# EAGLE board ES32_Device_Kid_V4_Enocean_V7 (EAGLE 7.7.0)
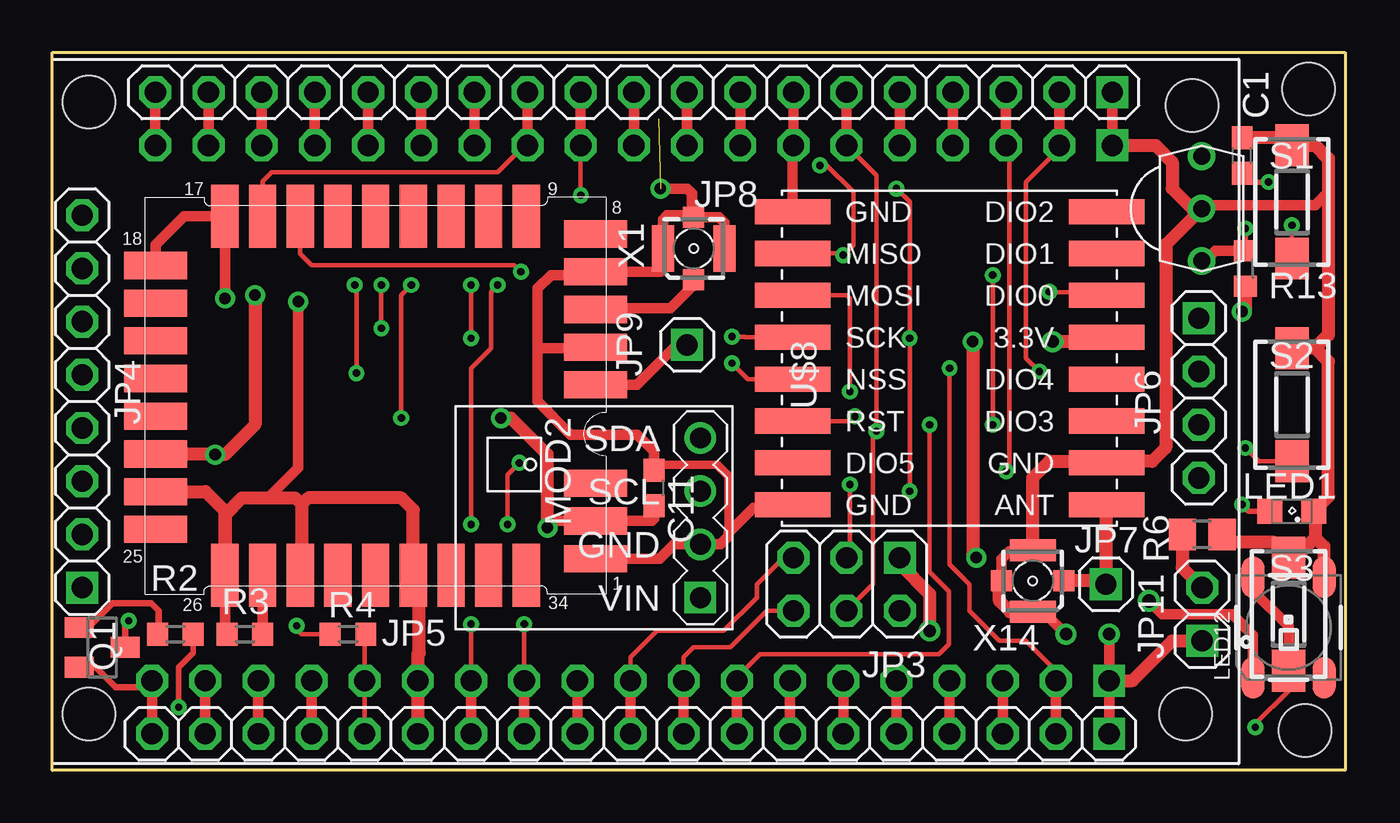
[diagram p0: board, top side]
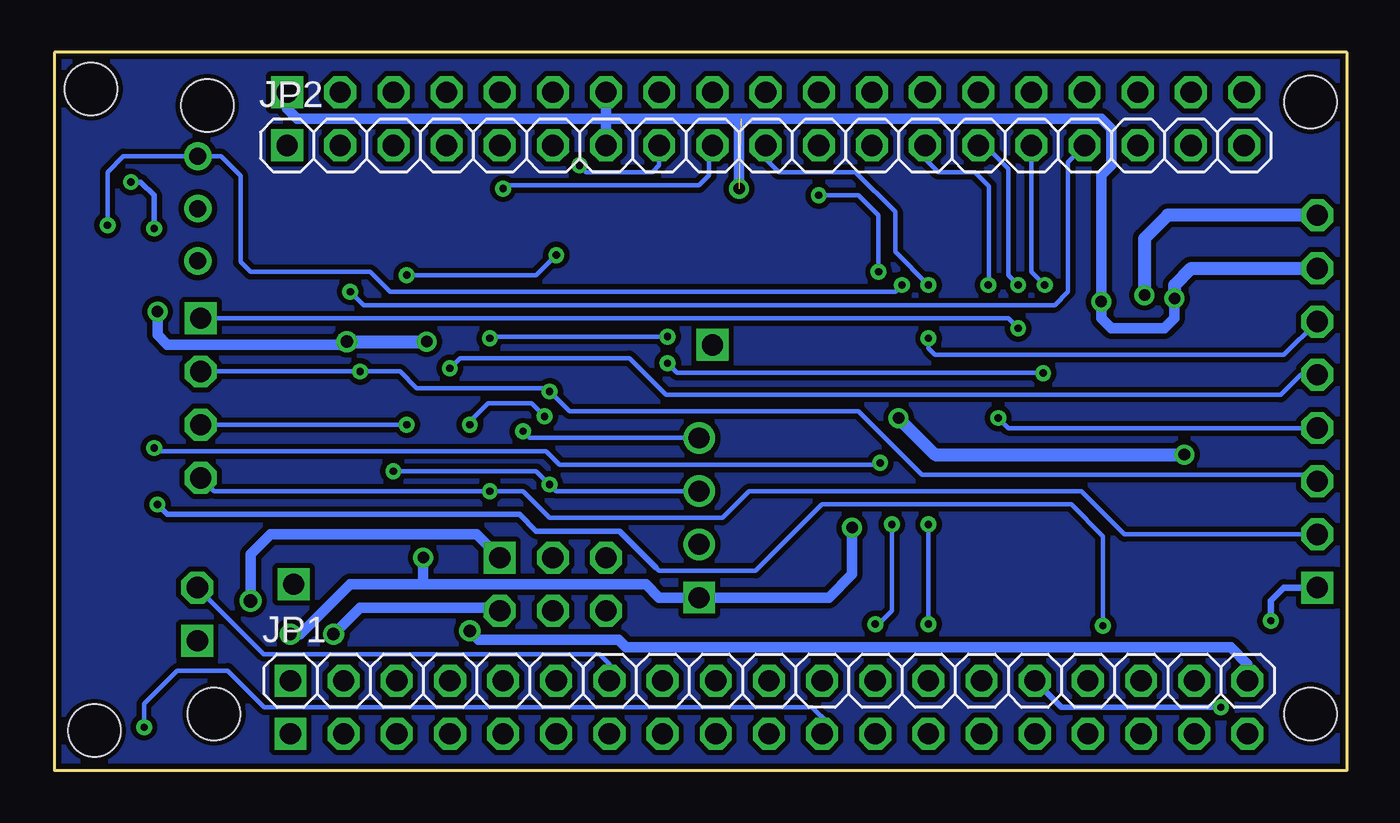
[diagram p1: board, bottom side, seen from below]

Size 61.75 x 34.29 mm. Coordinates in mm from the lower left corner, seen from the top.
Outline: 0,34.29 61.75,34.29 61.75,0 0,0 0,34.29
Copper layers (1*16): Top 0.035mm / dielectric 1.5mm / Bottom 0.035mm
Design rules "default *": minimum track width 6mil, minimum drill 0.35mm, track to track 6mil, track to pad 6mil, pad to pad 6mil, via to via 6mil, smd to smd 6mil, copper to edge 10mil, drill to drill 6mil, minimum pad ring 10mil, minimum via ring 8mil, stop-mask expansion 4mil, vias tented up to drill 0mil, thermal gap 10mil
Net classes: 1 pwr: width 0.25 mm, clearance 0.152 mm to class 0, clearance 0.152 mm
Holes 2.5 mm at 54.13,2.7 59.85,1.91 60.01,32.54 1.75,31.91 54.45,31.75 1.75,2.7

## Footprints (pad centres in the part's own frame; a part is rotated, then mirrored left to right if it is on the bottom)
STM300(C)_TCM300(C)_FOOTPRINT = smd 3 x 1.3: 1 21.5,1.7; 2 21.5,3.5; 3 21.5,5.3; 4 21.5,10; 5 21.5,11.8; 6 21.5,13.6; 7 21.5,15.4; 8 21.5,17.2; 18 0.5,15.7; 19 0.5,13.9; 20 0.5,12.1; 21 0.5,10.3; 22 0.5,8.5; 23 0.5,6.7; 24 0.5,4.9; 25 0.5,3.1 | smd 1.3 x 3: 9 18.2,18.05; 10 16.4,18.05; 11 14.6,18.05; 12 12.8,18.05; 13 11,18.05; 14 9.2,18.05; 15 7.4,18.05; 16 5.6,18.05; 17 3.8,18.05; 26 3.8,0.9; 27 5.6,0.9; 28 7.4,0.9; 29 9.2,0.9; 30 11,0.9; 31 12.8,0.9; 32 14.6,0.9; 33 16.4,0.9; 34 18.2,0.9
C0603 = smd 1.1 x 1: 1 -0.85,0; 2 0.85,0
1X19-S = drill 1.016 square: 1 -22.86,0 | drill 1.016 octagon: 2 -20.32,0; 3 -17.78,0; 4 -15.24,0; 5 -12.7,0; 6 -10.16,0; 7 -7.62,0; 8 -5.08,0; 9 -2.54,0; 10 0,0; 11 2.54,0; 12 5.08,0; 13 7.62,0; 14 10.16,0; 15 12.7,0; 16 15.24,0; 17 17.78,0; 18 20.32,0; 19 22.86,0
2X03 = drill 1.016 square: 1 -2.54,-1.27 | drill 1.016 octagon: 2 -2.54,1.27; 3 0,-1.27; 4 0,1.27; 5 2.54,-1.27; 6 2.54,1.27
1X08-S = drill 1.016 square: 1 -8.89,0 | drill 1.016 octagon: 2 -6.35,0; 3 -3.81,0; 4 -1.27,0; 5 1.27,0; 6 3.81,0; 7 6.35,0; 8 8.89,0
1X04-S = drill 1.016 square: 1 -3.81,0 | drill 1.016 octagon: 2 -1.27,0; 3 1.27,0; 4 3.81,0
1X01-S = drill 1.016 square: 1 0,0
1X02-S = drill 1.016 square: 1 -1.27,0 | drill 1.016 octagon: 2 1.27,0
SML0805 = smd 1.2 x 1.2: A 1.05,0; C -1.05,0
WS2812B = smd 2 x 1.1: 1 -2.4,1.7; 2 -2.4,-1.7; 3 2.4,-1.7; 4 2.4,1.7
TEMP-HUM-PRES-BME280 = drill 1 square: 1 -5.08,3.81 | drill 1: 2 -5.08,1.27; 3 -5.08,-1.27; 4 -5.08,-3.81
SOT23 = smd 1 x 1.4: 1 -0.95,-1.1; 2 0.95,-1.1; 3 0,1.1
R0603 = smd 1 x 1.1: 1 -0.85,0; 2 0.85,0
R0805 = smd 1.3 x 1.5: 1 -0.95,0; 2 0.95,0
DTSM-3 = smd 2 x 1.6: 1 -2.7,0; 2 2.7,0
TSOP18XX = drill 0.813: GND -0.001,-0.027; OUT -2.501,-0.027; VCC 2.499,-0.027
WIRELESS-LORA-RFM95W#SMD = smd 3.6 x 1.2: A1 -7.5,7; A2 -7.5,5; A3 -7.5,3; A4 -7.5,1; A5 -7.5,-1; A6 -7.5,-3; A7 -7.5,-5; A8 -7.5,-7; B1 7.5,7; B2 7.5,5; B3 7.5,3; B4 7.5,1; B5 7.5,-1; B6 7.5,-3; B7 7.5,-5; B8 7.5,-7
734120110 = smd 1 x 1: 1 0,-1.5; S@1 0,1.5 | smd 1.05 x 2.2: S@2 -1.475,0; S@3 1.475,0

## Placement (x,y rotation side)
BRD1  STM300(C)_TCM300(C)_DEVICE  [STM300(C)_TCM300(C)_FOOTPRINT]  4.45,8.41 0 top
C1  100n  [C0603]  56.83,29.37 90 top
C11  100nF  [C0603]  28.73,13.49 270 top
JP1  [1X19-S]  27.62,4.29 0 bottom
JP2  [1X19-S]  27.78,29.84 0 bottom
JP3  [2X03]  37.94,8.89 180 top
JP4  [1X08-S]  1.43,17.62 90 top
JP5  [1X19-S]  27.62,1.75 180 top
JP6  [1X04-S]  54.77,17.78 270 top
JP7  [1X01-S]  50.32,8.89 0 top
JP8  [1X19-S]  27.78,32.38 180 top
JP9  [1X01-S]  30.32,20.32 0 top
JP11  [1X02-S]  54.93,7.46 90 top
LED1  [SML0805]  59.21,12.38 180 top
LED12  WS2812B  [WS2812B]  59.05,6.83 90 top
MOD2  TEMP-HUM-PRES-BME280  [TEMP-HUM-PRES-BME280]  25.88,12.06 180 top
Q1  BSS84/IRLML2244  [SOT23]  2.38,5.87 270 top
R2  2K2  [R0603]  5.87,6.51 180 top
R3  10K / 0603  [R0603]  9.21,6.51 0 top
R4  470R  [R0603]  14.13,6.51 0 top
R6  470R  [R0805]  54.93,11.27 180 top
R13  100R  [R0603]  56.99,23.97 270 top
S1  DTSM-3  [DTSM-3]  59.21,27.15 270 top
S2  DTSM-3  [DTSM-3]  59.21,17.46 270 top
S3  DTSM-3  [DTSM-3]  59.05,7.46 270 top
U$5  TSOP1833  [TSOP18XX]  54.93,26.83 270 top
U$8  WIRELESS-LORA-RFM95W#SMD  [WIRELESS-LORA-RFM95W#SMD]  42.86,19.68 0 top
X1  734120110  [734120110]  30.64,24.92 0 top
X14  734120110  [734120110]  46.83,9.05 90 top

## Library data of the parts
BRD1 = STM300_TCM300_Eagle_Footprint
C1 = rcl; SPICEPREFIX: C
C11 = rcl@1
JP1-JP9 JP11 = pinhead-2
LED1 = led
LED12 = WS2812
MOD2 = diy-modules2
Q1 = transistor-small-signal
R2-R4 R6 R13 = rcl; SPICEPREFIX: R
S1-S3 = switch-tact
U$5 = tsop
U$8 = diy-modules
X1 X14 = con-coax

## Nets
+3V3: BRD1.2 BRD1.23 C11.2 JP1.1 JP4.8 JP5.1 JP11.1 MOD2.1 R13.2 U$8.B4
+5V: JP1.19 JP3.1 JP5.19 LED12.1 Q1.2
ENORES: BRD1.27 R3.2
GND [pwr]: BRD1.1 BRD1.5 BRD1.7 BRD1.17 BRD1.18 BRD1.24 BRD1.26 BRD1.28 BRD1.31 C1.2 C11.1 JP1.14 JP2.1 JP2.7 JP3.2 JP4.7 JP5.14 JP8.1 JP8.7 LED1.C LED12.3 MOD2.2 R3.1 R6.1 S1.1 S2.1 S3.1 U$5.GND U$8.A1 U$8.A8 U$8.B7 X1.S@1 X1.S@2 X1.S@3 X14.S@1 X14.S@2 X14.S@3
GP00_T1: JP2.14 JP6.1 JP8.14
GP01_TX0*: JP2.4 JP8.4
GP02_T2: JP2.15 JP8.15 U$8.A5
GP03_RX0*: JP2.5 JP8.5
GP04_T0: JP2.13 JP4.4 JP8.13
GP05_SS: JP2.10 JP4.6 JP8.10
GP06_SPI*: JP2.19 JP8.19
GP07_SPI*: JP2.18 JP8.18
GP08_SPI*: JP2.17 JP8.17
GP9_SPI*: JP1.16 JP5.16
GP10_SPI*: JP1.17 JP5.17
GP11_SPI*: JP1.18 JP5.18
GP12_T5: JP1.13 JP5.13 S1.2 U$5.OUT
GP13_ADC2-4: JP1.15 JP5.15 R2.1 R4.2
GP14_T6: JP1.12 JP5.12 S2.2
GP15_T3: JP2.16 JP8.16 U$8.B3
GP16_RX2: BRD1.16 JP2.12 JP8.12
GP17_TX2: BRD1.15 JP2.11 JP8.11
GP18_CLK: JP2.9 JP4.2 JP6.4 JP8.9 U$8.A4
GP19_MISO: JP2.8 JP6.3 JP8.8 U$8.A2
GP21_I2C-SDA: JP2.6 JP3.4 JP8.6 MOD2.4
GP22_I2C-CLK: JP2.3 JP3.3 JP8.3 MOD2.3
GP23_MOSI: JP2.2 JP4.3 JP6.2 JP8.2 U$8.A3
GP25_DAC1: JP1.9 JP3.6 JP5.9
GP26_DAC2: JP1.10 JP3.5 JP5.10
GP27_T7: JP1.11 JP5.11 LED12.4 S3.2
GP32_T9: JP1.7 JP5.7 JP11.2 R6.2
GP33_T8: JP1.8 JP5.8 U$8.A6
GP34_IN*: JP1.5 JP5.5
GP35_IN*: JP1.6 JP5.6
GP36_IN*: JP1.3 JP5.3
GP39_IN*: JP1.4 JP5.4
N$1: LED1.A R4.1
N$2: JP4.1 Q1.3
N$3: Q1.1 R2.2
N$8: JP7.1 U$8.B8 X14.1
N$9: C1.1 R13.1 U$5.VCC
RESET: JP1.2 JP4.5 JP5.2
RF50R: BRD1.6 X1.1
RFWIPE: BRD1.4 JP9.1

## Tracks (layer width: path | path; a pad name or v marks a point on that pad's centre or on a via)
+3V3  (via drill 0.55, 0.6)
  Top 0.508: U$8.B4 49.58,20.68 | v50.48,6.51 JP1.1 JP5.1 | v23.65,11.59 23.98,11.91 BRD1.2 28.64,11.91 28.73,12.01 C11.2 | 7.75,15.11 v7.78,15.08
  Top 0.61: JP1.1 51.59,4.29 53.5,6.19 JP11.1 | R13.2 56.99,22.07 v56.83,21.91 | 49.58,20.68 49.37,20.48 v47.78,20.48 | v43.97,20.48 43.97,10.32 v44.13,10.16 | v23.65,11.59 23.65,15.08 21.91,16.83 v21.43,16.83 | BRD1.23 7.75,15.11 | v9.68,22.7 9.68,16.51 8.26,15.08 v7.78,15.08
  Bottom 0.508: 44.13,8.89 33.5,8.89 32.86,8.26 MOD2.1 24.77,8.26 23.65,9.37 v23.65,11.59 | 44.13,8.89 47.62,8.89 50.01,6.51 v50.48,6.51 | v47.78,20.48 47.94,20.32 56.36,20.32 56.83,20.8 v56.83,21.91 | v44.13,10.16 44.13,8.89
  Bottom 0.61: v47.78,20.48 v43.97,20.48 | JP4.8 8.57,26.51 9.68,25.4 v9.68,22.7 | v21.43,16.83 19.68,15.08 v7.78,15.08
+5V  (via drill 0.6, 0.64)
  Top 0.305: Q1.2 2.06,4.92 3.02,3.97 4.45,3.97 JP1.19
  Top 0.508: JP5.19 JP1.19 | LED12.1 57.35,6.46 56.36,7.46 53.02,7.46 v52.39,8.1
  Top 0.61: v41.91,6.67 41.91,8.41 40.48,9.84 JP3.1
  Bottom 0.508: v41.91,6.67 41.48,6.24 34.82,6.24 34.45,5.87 5.56,5.87 4.76,5.08 JP1.19 | v52.39,8.1 52.39,10.32 51.44,11.27 41.59,11.27 JP3.1
ENORES
  Top 0.508: R3.2 10.06,9.3 BRD1.27
GD
  pour Bottom (isolate 0.254): 0.16,34.29 61.75,34.29 61.75,0.16 0,0.16 0,33.97
GND  (via drill 0.55, 0.6)  (1 unrouted)
  Top 0.406: C11.1 29,14.61 31.75,14.61 32.31,14.05 32.31,11.35 32.31,11.19
  Top 0.508: v48.42,6.51 47.35,7.57 X14.S@2 | BRD1.1 29,10.11 29.69,10.79 MOD2.2 31.91,10.79 32.31,11.19 | 32.31,11.35 33.5,12.54 35.22,12.54 U$8.A8 | C11.1 28.73,15.24 27.94,16.03 24.77,16.03 23.18,17.62 23.18,20.16 | 23.18,20.16 23.18,23.02 23.81,23.66 25.79,23.66 BRD1.7 29.05,23.81 29.16,23.93 X1.S@2 29.16,26.31 29.37,26.51 30.55,26.51 | JP2.1 JP8.1 | v11.75,22.38 11.75,14.45 10.32,13.02 | BRD1.18 4.95,25.11 6.3,26.46 BRD1.17 8.24,23.35 8.26,23.34 v8.26,22.54 | U$8.A1 35.36,29.81 JP2.7 JP8.7 | 30.55,26.51 X1.S@1 31.84,26.42 32.11,26.15 X1.S@3 | v29.05,27.78 30.32,27.78 30.55,27.55 30.55,26.51 | U$5.GND 55.06,26.99 60.33,26.99 60.96,27.62 | R3.1 8.24,6.62 BRD1.26 | BRD1.5 25.89,20.16 23.18,20.16 | X14.S@1 45.33,10.09 45.72,10.48 46.78,10.48 X14.S@3
  Top 0.61: C1.2 59.05,30.22 59.21,30.06 S1.1 60.32,29.85 60.96,29.21 60.96,27.62 60.96,20.8 60.33,20.16 | 60.33,20.16 S2.1 | R6.1 56.25,10.9 58.32,10.9 S3.1 59.37,10.16 60.33,11.11 | 60.33,11.11 60.33,12.32 LED1.C 60.96,13.08 60.96,19.53 60.33,20.16 | JP2.1 52.7,29.84 53.5,29.05 53.5,27.78 54.45,26.83 U$5.GND 53.18,25.11 53.18,15.4 52.55,14.76 50.44,14.76 U$8.B7 50.28,14.76 47.62,14.76 46.83,13.97 X14.S@3 | X14.S@2 45.77,7.57 45.24,8.1 45.24,8.96 X14.S@1 | BRD1.24 7.32,13.31 8.26,12.38 8.26,9.32 BRD1.26 8.24,12.21 9.05,13.02 10.32,13.02 11.59,13.02 11.91,12.7 | 11.91,12.7 11.91,9.38 BRD1.28 | 11.91,12.7 12.22,13.02 16.67,13.02 17.25,12.44 BRD1.31 17.52,9.04 17.52,5.61 17.46,5.55 JP1.14 JP5.14 | LED12.3 60.76,10.68 60.33,11.11
  Bottom 0.508: JP3.2 40.64,7.78 47.15,7.78 v48.42,6.51 | JP8.1 50.64,31.59 50.16,31.11 35.56,31.11 35.4,31.27 | JP2.7 35.4,31.27 | 35.4,31.27 JP8.7 | 35.4,31.27 35.24,31.11 29.11,31.11 29.05,31.06 v29.05,27.78 | 28.95,31.11 11.75,31.11 11.27,30.64 11.27,28.89 11.75,28.42 v11.75,22.38 11.75,21.59 11.27,21.11 8.73,21.11 8.26,21.59 v8.26,22.54
  Bottom 0.61: JP4.7 7.46,23.97 8.26,23.18 v8.26,22.54
GP00_T1  (via drill 0.35)
  Top 0.203: v15.72,23.18 v15.72,21.11
  Top 0.508: JP8.14 JP2.14
  Bottom 0.203: JP6.1 16.19,21.59 v15.72,21.11 | v15.72,23.18 16.19,23.65 16.19,28.73 17.3,29.84 JP2.14
GP01_TX0*
  Top 0.508: JP8.4 JP2.4
GP02_T2  (via drill 0.35)
  Top 0.203: U$8.A5 33.23,18.68 v32.46,19.45 | v14.45,23.18 14.53,23.1 v14.53,18.97
  Top 0.508: JP8.15 JP2.15
  Bottom 0.203: v32.46,19.45 32,18.99 14.51,18.99 v14.53,18.97 | JP2.15 15.08,23.81 v14.45,23.18
GP03_RX0*
  Top 0.508: JP8.5 JP2.5
GP04_T0  (via drill 0.35)
  Top 0.203: v17.14,23.18 16.67,22.7 v16.67,16.83
  Top 0.508: JP8.13 JP2.13
  Bottom 0.203: v16.67,16.83 16.19,16.35 JP4.4 | v17.14,23.18 17.11,23.22 17.11,27.9 17.78,28.57 19.53,28.57 20.16,29.21 JP2.13
GP05_SS  (via drill 0.35)
  Top 0.203: v20,23.18 v20,20.64
  Top 0.508: JP8.10 JP2.10
  Bottom 0.203: v20,20.64 20,20.16 19.68,19.84 3.02,19.84 JP4.6 | v20,23.18 21.59,24.77 21.59,26.67 23.5,28.57 27.15,28.57 27.78,29.21 JP2.10
GP06_SPI*
  Top 0.508: JP2.19 JP8.19
GP07_SPI*
  Top 0.508: JP8.18 JP2.18
GP08_SPI*
  Top 0.508: JP8.17 JP2.17
GP9_SPI*
  Top 0.508: JP1.16 JP5.16
GP10_SPI*
  Top 0.508: JP5.17 JP1.17
GP11_SPI*
  Top 0.508: JP5.18 JP1.18
GP12_T5  (via drill 0.35)
  Top 0.203: S1.2 v59.21,26.04 | JP1.13 v20,6.99 | v21.27,23.18 20.95,22.86 20.95,20.16 20,19.21 v20,11.75
  Top 0.508: JP5.13 JP1.13
  Bottom 0.203: v59.21,26.04 59.21,28.57 58.46,29.33 U$5.OUT 53.79,29.33 52.86,28.4 52.86,24.29 52.39,23.81 46.67,23.81 45.72,22.86 21.59,22.86 v21.27,23.18 | v20,11.75 v20,6.99
GP13_ADC2-4  (via drill 0.35)
  Top 0.203: R4.2 14.92,6.45 JP1.15 JP5.15
  Top 0.254: R2.1 6.72,5.61 6.03,4.92 v6.03,3.02
  Bottom 0.254: v6.03,3.02 13.65,3.02 JP1.15
GP14_T6  (via drill 0.35)
  Top 0.203: S2.2 57.63,14.76 v56.99,15.4 | JP1.12 v22.54,6.99 | v21.75,11.75 21.75,14.13 v22.3,14.68
  Top 0.508: JP5.12 JP1.12
  Bottom 0.203: v56.99,15.4 56.83,15.24 38.26,15.24 37.62,14.61 22.38,14.61 v22.3,14.68 | v22.54,6.99 22.38,6.99 21.75,7.62 v21.75,11.75
GP15_T3  (via drill 0.35)
  Top 0.203: U$8.B3 50.2,22.84 47.8,22.84 47.78,22.86 v47.62,22.86
  Top 0.508: JP8.16 JP2.16
  Bottom 0.203: v47.62,22.86 46.99,22.23 13.97,22.23 13.34,22.86 13.34,29.05 JP2.16
GP16_RX2
  Top 0.203: BRD1.16 10.04,28.14 10.48,28.57 21.27,28.57 22.7,30
  Top 0.508: JP8.12 22.7,30 JP2.12
GP17_TX2  (via drill 0.35)
  Top 0.203: BRD1.15 11.85,24.67 12.38,24.13 22.07,24.13 v22.38,23.81 | v25.24,27.46 25.24,30
  Top 0.508: JP8.11 25.24,30 JP2.11
  Bottom 0.203: v22.38,23.81 22.38,26.51 23.34,27.46 v25.24,27.46
GP18_CLK  (via drill 0.35)
  Top 0.203: v40.32,27.78 40.96,27.15 v40.96,20.64 v40.96,13.34 | U$8.A4 33.07,20.68 33.1,20.72 v32.46,20.72
  Top 0.508: JP8.9 JP2.9
  Bottom 0.203: JP6.4 54.13,13.34 v40.96,13.34 39.37,13.34 38.1,12.06 29.84,12.06 28.57,13.34 12.7,13.34 10.64,11.27 JP4.2 | JP2.9 30.48,29.69 30.48,28.42 30.96,27.94 40.16,27.94 v40.32,27.78 | v32.46,20.72 40.88,20.72 v40.96,20.64
GP19_MISO  (via drill 0.35)
  Top 0.203: v36.67,28.89 36.99,28.89 38.26,27.62 38.26,25.08 v37.78,24.61 37.7,24.68 U$8.A2 | v44.93,23.65 v44.93,16.51
  Top 0.508: JP8.8 JP2.8
  Bottom 0.203: JP6.3 v44.93,16.51 | v36.67,28.89 36.35,28.57 33.18,28.57 32.86,28.89 JP2.8 | v44.93,23.65 38.73,23.65 v37.78,24.61
GP21_I2C-SDA  (via drill 0.35)
  Top 0.203: 38.02,29.77 39.37,28.42 v39.37,16.19 39.21,16.03 39.21,8.89 JP3.4
  Top 0.508: JP8.6 JP2.6 38.02,29.77
  Bottom 0.203: MOD2.4 39.05,15.88 v39.37,16.19
GP22_I2C-CLK  (via drill 0.35)
  Top 0.203: JP2.3 45.72,29.69 45.72,14.45 v45.56,14.29 | v38.1,13.65 38.1,10.32 JP3.3
  Top 0.508: JP8.3 JP2.3
  Bottom 0.203: MOD2.3 37.78,13.34 v38.1,13.65 38.73,14.29 v45.56,14.29
GP23_MOSI  (via drill 0.35)
  Top 0.203: JP2.2 48.1,29.69 46.51,28.1 46.51,19.68 v47.15,19.05 | U$8.A3 37.96,22.68 38.1,22.54 v38.1,18.1
  Top 0.508: JP8.2 JP2.2
  Bottom 0.203: JP6.2 v47.15,19.05 45.24,19.05 44.45,18.26 38.26,18.26 v38.1,18.1 37.15,17.14 23.34,17.14 20.32,14.13 1.75,14.13 JP4.3
GP25_DAC1
  Top 0.203: JP1.9 30.16,5.4 30.64,5.87 32.38,5.87 34.13,7.62 JP3.6
  Top 0.508: JP1.9 JP5.9
GP26_DAC2
  Top 0.203: JP1.10 27.62,4.45 27.62,5.4 28.89,6.67 32.07,6.67 33.66,8.26 33.66,8.89 34.92,10.16 JP3.5
  Top 0.508: JP5.10 27.62,4.45
GP27_T7  (via drill 0.35)
  Top 0.203: S3.2 59.05,3.81 57.47,2.22 v57.47,2.06
  Top 0.508: JP5.11 JP1.11 | LED12.4 57.35,8.59 59.05,6.89 S3.2
  Bottom 0.203: v57.47,2.06 57.47,3.17 55.88,4.76 53.48,4.76 51.73,3.02 25.56,3.02 24.77,2.22 24.77,2.06 JP5.11
GP32_T9
  Top 0.508: JP1.7 JP5.7
  Top 0.61: R6.2 53.98,9.68 JP11.2
  Bottom 0.203: JP1.7 35.24,5.08 35.72,5.56 51.75,5.56 JP11.2
GP33_T8  (via drill 0.35)
  Top 0.203: JP1.8 32.7,4.45 33.81,5.56 42.36,5.56 42.84,6.03 42.84,8.56 41.91,9.48 v41.91,16.51 | U$8.A6 38.12,16.68 v38.34,16.91
  Top 0.508: JP1.8 JP5.8
  Bottom 0.203: v38.34,16.91 38.97,17.54 41.04,17.54 41.91,16.67 v41.91,16.51
GP34_IN*
  Top 0.508: JP1.5 JP5.5
GP35_IN*
  Top 0.508: JP1.6 JP5.6
GP36_IN*
  Top 0.508: JP1.3 JP5.3
GP39_IN*
  Top 0.508: JP1.4 JP5.4
N$1  (via drill 0.35)
  Top 0.203: R4.1 11.91,6.51 11.51,6.91 v11.67,6.91
  Top 0.254: LED1.A 57.15,12.38 v56.83,12.7
  Bottom 0.203: 33.02,9.68 32.86,9.53 28.26,9.53 25.08,12.7 13.18,12.7 11.67,11.19 v11.67,6.91
  Bottom 0.254: v56.83,12.7 56.36,12.22 39.53,12.22 38.73,11.43 34.77,11.43 33.02,9.68
N$2  (via drill 0.35)
  Top 0.305: Q1.3 3.48,6.97 v3.65,7.14
  Bottom 0.305: v3.65,7.14 3.65,8.1 3.02,8.73 JP4.1
N$3
  Top 0.305: Q1.1 1.44,6.99 1.89,6.99 2.89,7.99 4.71,7.99 5.08,7.62 5.08,6.57 R2.2
N$8
  Top 0.61: U$8.B8 50.32,12.65 JP7.1 50.16,9.05 X14.1
N$9  (via drill 0.35)
  Top 0.254: v58.1,28.1 57.25,28.1 C1.1 | v56.99,25.88 R13.1
  Top 0.508: U$5.VCC 55.06,24.33 55.55,24.82 R13.1
  Bottom 0.254: v58.1,28.1 57.63,28.1 56.99,27.46 v56.99,25.88
RESET  (via drill 0.35)
  Top 0.203: JP1.2 47.94,4.76 46.51,6.19 45.24,6.19 43.81,7.62 43.81,8.89 42.86,9.84 v42.86,19.21
  Top 0.508: JP1.2 JP5.2
  Bottom 0.203: JP4.5 2.22,18.89 3.17,17.94 32.54,17.94 34.29,19.68 42.39,19.68 v42.86,19.21
RF50R
  Top 0.508: BRD1.6 26,22.07 29.53,22.07 30.64,23.18 X1.1
RFWIPE
  Top 0.508: BRD1.4 27.94,18.41 29.84,20.32 JP9.1

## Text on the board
Document: +3V3 | IR | GND | SEL/GP05 | RES | SEL/GP00 | CMD/GP04 | MOSI | MOSI | MISO | SPI CLK | SPI CLK | LED | LDR | SYS LED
